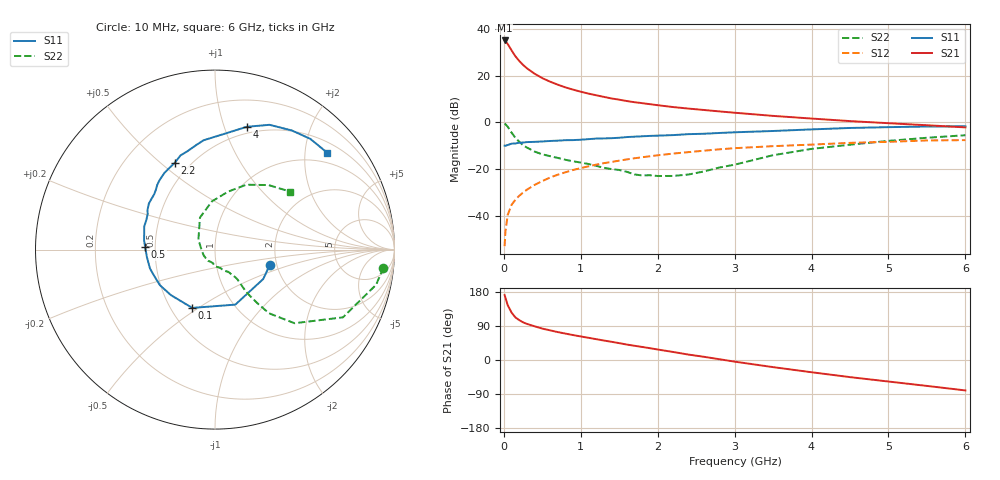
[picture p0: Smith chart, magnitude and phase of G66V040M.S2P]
! SIEMENS Small Signal Semiconductors
! BFG193
! Si NPN RF Bipolar Junction Transistor in SOT223
! VCE = 6 V  IC = 40 mA
! Common Emitter S-Parameters:  August  1996
# GHz  S  MA  R  50
!  f  S11  S21  S12  S22
! GHz  MAG  ANG  MAG  ANG  MAG  ANG  MAG  ANG
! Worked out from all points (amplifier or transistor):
!   36 points, 10 MHz to 6 GHz, reference 50 ohm
!   highest |S21| = 35.2 dB at 10 MHz (marker M1)
!   |S21| within 3 dB of that: start of sweep to 77.35 MHz
!   unconditionally stable (mu >= 1): 491.9 MHz to 2.379 GHz
!   at 250 MHz: K = 0.88, MSG = 27.4 dB, |S12| = -30.1 dB
!   at 1.4 GHz: K = 1.05, MAG = 12.3 dB, |S12| = -17.0 dB
!   at 6 GHz: K = 0.89, MSG = 2.7 dB, |S12| = -7.6 dB
!   S11 on the Smith chart (normalised r, x): 10 MHz: 1.84, -0.35; 100 MHz: 0.64, -0.47; 500 MHz: 0.44, +0.01; 2.2 GHz: 0.41, +0.56; 4 GHz: 0.44, +1.19; 6 GHz: 0.73, +2.49
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0.01  0.317 -15.7  57.36 171.5  0.0022 87.8  0.9435 -6.1
0.02  0.3148 -31.4  55.66 164.7  0.0044 81.9  0.9188 -12.3
0.05  0.3268 -69.7  48.19 144.9  0.0103 71.7  0.8066 -27.9
0.1  0.3487 -111.3  35.23 125.2  0.0169 66.4  0.6038 -42.8
0.15  0.3531 -134.1  26.28 112.4  0.0218 65.3  0.4652 -49.7
0.2  0.3653 -147.1  20.86 105.2  0.0265 66.2  0.3837 -51.6
0.25  0.3689 -156.3  17.11 99.4  0.0312 65.8  0.3233 -52.9
0.3  0.3773 -163.8  14.49 95.3  0.0359 67.1  0.2877 -53.6
0.4  0.3817 -173.7  11.06 88.9  0.0455 67.5  0.236 -53.3
0.5  0.3892 178.1  8.909 82.9  0.0549 67.1  0.2059 -53.0
0.6  0.3988 172.4  7.494 78.3  0.0654 66.3  0.1882 -53.9
0.7  0.4051 166.7  6.456 73.7  0.0752 65.1  0.1728 -55.8
0.8  0.4147 162.0  5.643 69.7  0.0849 63.5  0.1574 -57.4
1.1  0.4363 149.5  4.146 58.6  0.1139 58.5  0.1278 -66.9
1.6  0.484 131.6  2.867 40.7  0.1603 48.1  0.0867 -93.2
2.2  0.533 114.9  2.133 21.2  0.2137 34.7  0.0708 -153.5
2.8  0.5922 100.1  1.721 2.1  0.2638 20.9  0.1072 149.5
3.5  0.6531 84.1  1.378 -18.8  0.3088 3.9  0.1974 115.1
4  0.7068 75.5  1.208 -32.3  0.3331 -5.9  0.2695 93.6
4.5  0.7587 66.4  1.065 -45.2  0.3633 -16.0  0.3314 77.2
5.5  0.814 49.3  0.868 -68.4  0.4095 -39.3  0.4673 50.3
6  0.8259 40.9  0.781 -80.3  0.4158 -52.7  0.53 37.5
